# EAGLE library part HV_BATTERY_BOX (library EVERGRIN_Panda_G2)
HV battery box
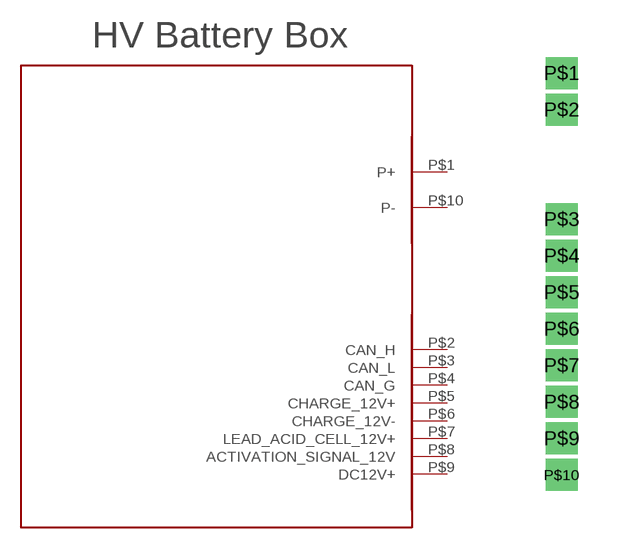
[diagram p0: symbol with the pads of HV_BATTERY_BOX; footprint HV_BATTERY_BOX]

Designator prefix -

## HV_BATTERY_BOX  [HV_BATTERY_BOX]
P$1  P+  pwr
P$2  CAN_H
P$3  CAN_L
P$4  CAN_G
P$5  CHARGE_12V+
P$6  CHARGE_12V-
P$7  LEAD_ACID_CELL_12V+
P$8  ACTIVATION_SIGNAL_12V
P$9  DC12V+
P$10  P-  pwr

## Footprint HV_BATTERY_BOX (pad centres in mm)
drill 0.6 square: P$1 0,17.78; P$2 0,16.51; P$3 0,12.7; P$4 0,11.43; P$5 0,10.16; P$6 0,8.89; P$7 0,7.62; P$8 0,6.35; P$9 0,5.08; P$10 0,3.81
